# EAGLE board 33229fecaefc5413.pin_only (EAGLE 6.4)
REV: G

Size 35.56 x 17.78 mm. Coordinates in mm from the lower left corner, seen from the top.
Outline: 0,6.35 0,1.27 arc90 1.27,0 34.29,0 arc90 35.56,1.27 35.56,16.51 arc90 34.29,17.78 1.27,17.78 arc90 0,16.51 0,11.68 0.51,11.18 0.51,6.86 0,6.35
Copper layers (1*16): Top 0.035mm / dielectric 1.5mm / Bottom 0.035mm
Design rules "adafruit *": minimum track width 8mil, minimum drill 15.5mil, track to track 8mil, track to pad 8mil, pad to pad 8mil, via to via 8mil, smd to smd 8mil, copper to edge 10mil, drill to drill 8mil, minimum pad ring 10mil, minimum via ring 8mil, stop-mask expansion 2mil, vias tented up to drill 20mil, thermal gap 10mil

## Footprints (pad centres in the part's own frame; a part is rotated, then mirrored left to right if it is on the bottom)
0603-NO = smd 1.075 x 1: 1 -0.85,0; 2 0.85,0
0805-NO = smd 1.24 x 1.5: 1 -0.95,0; 2 0.95,0
SOD-123FL = smd 0.91 x 1.22: A 1.637,0; C -1.637,0
SOT23-5 = smd 0.69 x 0.99: 1 -0.95,-1.29; 2 0,-1.29; 3 0.95,-1.29; 4 0.95,1.3; 5 -0.95,1.3
1X05_ROUND_70 = drill 1 pad 1.778: 1 -5.08,0; 2 -2.54,0; 3 0,0; 4 2.54,0; 5 5.08,0
1X14_ROUND70 = drill 1 pad 1.676: 1 -16.51,0; 2 -13.97,0; 3 -11.43,0; 4 -8.89,0; 5 -6.35,0; 6 -3.81,0; 7 -1.27,0; 8 1.27,0; 9 3.81,0; 10 6.35,0; 11 8.89,0; 12 11.43,0; 13 13.97,0; 14 16.51,0
CHIPLED_0805_NOOUTLINE = smd 1.2 x 1.2: A 0,-1.05; C 0,1.05
APA102_2020 = smd 0.7 x 0.35: 1 -0.95,-0.75; 2 -0.95,0; 3 -0.95,0.75; 4 0.95,0.75; 5 0.95,0; 6 0.95,-0.75
KMR2 = smd 1 x 1: 1 2,0.8; 2 2,-0.8; 3 -2,0.8; 4 -2,-0.8
USON8 = smd 0.35 x 0.25: 1 -1.2,0.75; 2 -1.2,0.25; 3 -1.2,-0.25; 4 -1.2,-0.75; 5 1.2,-0.75; 6 1.2,-0.25; 7 1.2,0.25; 8 1.2,0.75
SOT23-5' = smd 0.55 x 1.2: 1 -0.95,-1.3; 2 0,-1.3; 3 0.95,-1.3; 4 0.95,1.3; 5 -0.95,1.3
TQFN48_7MM = smd 0.25 x 0.75: 1 -2.75,-3.475; 2 -2.25,-3.475; 3 -1.75,-3.475; 4 -1.25,-3.475; 5 -0.75,-3.475; 6 -0.25,-3.475; 7 0.25,-3.475; 8 0.75,-3.475; 9 1.25,-3.475; 10 1.75,-3.475; 11 2.25,-3.475; 12 2.75,-3.475; 25 2.75,3.475; 26 2.25,3.475; 27 1.75,3.475; 28 1.25,3.475; 29 0.75,3.475; 30 0.25,3.475; 31 -0.25,3.475; 32 -0.75,3.475; 33 -1.25,3.475; 34 -1.75,3.475; 35 -2.25,3.475; 36 -2.75,3.475 | smd 0.75 x 0.25: 13 3.475,-2.75; 14 3.475,-2.25; 15 3.475,-1.75; 16 3.475,-1.25; 17 3.475,-0.75; 18 3.475,-0.25; 19 3.475,0.25; 20 3.475,0.75; 21 3.475,1.25; 22 3.475,1.75; 23 3.475,2.25; 24 3.475,2.75; 37 -3.475,2.75; 38 -3.475,2.25; 39 -3.475,1.75; 40 -3.475,1.25; 41 -3.475,0.75; 42 -3.475,0.25; 43 -3.475,-0.25; 44 -3.475,-0.75; 45 -3.475,-1.25; 46 -3.475,-1.75; 47 -3.475,-2.25; 48 -3.475,-2.75 | smd 4.7 x 4.7: THERMAL 0,0
FIDUCIAL_1MM = smd 1 x 1: 1 0,0
JSTPH2 = smd 1 x 4.6: 1 -1,-3.7; 2 1,-3.7 | smd 1.6 x 3.4: NC1 -3.4,1.5; NC2 3.4,1.5
4UCONN_20329_V2 = smd 1 x 2: BASE@1 -0.75,-2; BASE@2 0.75,-2 | smd 0.4 x 1.35: D+ 0,0.775; D- -0.65,0.775; GND 1.3,0.775; ID 0.65,0.775; VBUS -1.3,0.775 | drill 0.8 pad 1.143 offset: SPRT@1 -3.3,0.9; SPRT@2 3.3,0.9 | drill 0.9 pad 2.413 square: SPRT@3 -3.6,-1.9; SPRT@4 3.6,-1.9 | hole 0.7: -1.95,0; 1.95,0

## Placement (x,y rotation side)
C1  1uF  [0603-NO]  11.91,9.27 180 top
C5  1uF  [0603-NO]  27.24,6.03 0 top
C6  10µF  [0805-NO]  8.58,9.31 0 top
C7  1uF  [0603-NO]  16.27,13.1 180 top
C8  10µF  [0805-NO]  11.94,7.73 180 top
C14  1uF  [0603-NO]  11.35,4.03 0 top
D1  MBR120  [SOD-123FL]  8.89,13.59 180 top
D2  MBR120  [SOD-123FL]  8.89,11.81 180 top
IC1  74HCT1G125  [SOT23-5]  26.92,12.13 0 top
JP1  [1X05_ROUND_70]  34.29,8.89 90 top
JP2  [1X14_ROUND70]  17.78,16.51 0 top
JP4  [1X14_ROUND70]  17.78,1.27 180 top
L  RED  [CHIPLED_0805_NOOUTLINE]  30.38,12.36 270 top
L2  AP102-2020  [APA102_2020]  11.43,5.78 0 top
R1  100k  [0603-NO]  8.19,7.68 180 top
R2  100k  [0603-NO]  13.14,13.65 180 top
R7  2.2K  [0603-NO]  30.16,13.72 180 top
SW1  SPST_TACT-KMR2  [KMR2]  30.16,8.57 270 top
U1  flash  [USON8]  13.21,11.81 0 top
U2  AP2112K-3.3  [SOT23-5']  8.13,5.02 180 top
U$4  ATSAMD21G18  [TQFN48_7MM]  19.81,8.38 0 top
U$13  [PCBFEAT-REV-040]  3.75,8.89 0 bottom
U$14  [ITSYM0_TOP]  0,0 0 top
U$15  [ITSYM0_BOT]  35.56,0 0 bottom
U$34  FIDUCIAL_1MM  [FIDUCIAL_1MM]  30.42,9.02 270 top
U$35  FIDUCIAL_1MM  [FIDUCIAL_1MM]  2.27,2.99 270 top
X1  [JSTPH2]  3.56,8.89 270 bottom
X3  microUSB  [4UCONN_20329_V2]  4.45,8.89 270 top

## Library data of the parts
C1 C5-C7 C14 JP1 JP2 JP4 L L2 R1 R2 R7 U1 U2 U$4 U$13 X1 X3 = microbuilder
C8 = microbuilder; COMPANY: ADAFRUIT INDUSTRIES; DRAWN: KTOWN; REV: A
D1 D2 SW1 = adafruit
IC1 = 74xx-little-us
U$14 U$15 = silks
U$34 U$35 = microbuilder; BOM: EXCLUDE

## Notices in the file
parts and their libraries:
microbuilder: This work is placed in the public domain, and may be freely used for commercial and non-commercial work with the following conditions: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
